(* Logix 5000 AddOnInstructionDefinition export MCFG_Yaskawa; software revision 17.00 *)

TYPE Yaskawa_EIP_Servo :   // Yaskawa SigmaLogic Axis Structure
STRUCT
   O : Yaskawa_OUT_to_Servo;
   I : Yaskawa_IN_from_Servo;
   AOI_SB : Yaskawa_AOI_Status_Bits;
END_STRUCT
END_TYPE

TYPE Yaskawa_OUT_to_Servo :   // Structure of data sent out to the Yaskawa SigmaLogic controller
STRUCT
   b00_ServoOn : BOOL;   // Servo On
   b01_Stop : BOOL;   // Stops All Current Motion in Progress
   b02_Home : BOOL;   // Start Homing Process
   b03_MoveStart1 : BOOL;   // Start Current Motion
   b06_SuperImpose : BOOL;
   b07_ServoAlarmReset : BOOL;   // Servo Alarm Reset
   b08_ControllerAlarmReset : BOOL;   // SigmaLogic Alarm Reset
   b09_MoveStart2 : BOOL;   // Start Second Motion (Blended Move)
   b10_MoveAbort : BOOL;   // Abort Current Move
   b11_MovePause : BOOL;   // Pause Current Move
   b12_SeqPause : BOOL;   // Indexing Sequence Pause
   b13_SeqResume : BOOL;   // Indexing Sequence Resume
   b14_SeqCancel : BOOL;   // Indexing Sequence Cancel
   b15_AbsEncoderReset : BOOL;   // Absolute Encoder Reset
   b16_SeqStart : BOOL;   // Start Indexing Sequence
   b17_SeqEditSpeed : BOOL;   // Enter Edit Speed
   b18_SeqEditDistance : BOOL;   // Enter Distance Edit
   b19_PLSEnable : BOOL;   // Enable PLS execution
   b20_PLSActivateOutput1 : BOOL;   // Activate PLS output1 switch logic
   b21_PLSActivateOutput2 : BOOL;   // Activate PLS output2 switch logic
   b22_PLSActivateOutput3 : BOOL;   // Activate PLS output3 switch logic
   b23_PLSActivateOutput4 : BOOL;   // Activate PLS output4 switch logic
   b24_SetClock : BOOL;   // Set the remote controller clock with data provided by the PLC
   RebootController : BOOL;
   UseExternalEncoder : BOOL;   // Use External Encoder when executing MAHSP_Yaskawa
   b32_HeatbeatAnswer : BOOL;   // Heartbeat Answer
   BrakeBypassRequest : BOOL;
   TorqueLimit : DINT;
   TorqueRamp : DINT;
   HomeMethod : INT;
   HomeSpeed : DINT;
   HomeAccDec : DINT;   // Home Move Acceleration/Deceleration Rate
   HomeBackOffDistance : DINT;
   HomeCreepSpeed : DINT;
   HomeCreepDistanceLimit : DINT;
   HomeCreepTimeLimit : DINT;
   HomeOffsetDistance : DINT;
   HomeOffsetSpeed : DINT;
   HomePostion : DINT;
   HomeTorque : DINT;
   HomeInputNo : DINT;
   HomeApproachTimeLimit : DINT;
   HomeApproachDistLimit : DINT;
   HomeDirection : INT;
   HomeSwitchMode : INT;
   MoveType : INT;
   MoveDirection : INT;
   MoveAccel1 : DINT;
   MoveAccel2 : DINT;
   MoveDecel1 : DINT;
   MoveDecel2 : DINT;
   MoveSpeed1 : DINT;
   MoveSpeed2 : DINT;
   MoveDistance1 : DINT;
   MoveDistance2 : DINT;
   MovePosition1 : DINT;
   MovePosition2 : DINT;
   RegistrationDistance : DINT;
   GearNumerator : DINT;
   GearDenominator : DINT;
   SuperImposeDistance : DINT;
   Resolution : INT;
   RegistrationDirection : INT;
   TuningLevel : INT;
   SequenceStep : INT;   // Staring Sequence Step Number
   SequenceEditStep : INT;   // Sequence Step Number to Edit
   FlagCommandBits1 : DINT;   // Flag Commands. 1..64 are General Flags, Bits 0..31 correspond to Flag 1..32
   FlagCommandBits2 : DINT;   // Flag Commands cont. 1..64 are General Flags, Bits 0..31 correspond to Flag 33..64
   DigitalOutCommandBits : DINT;   // Digital Output commands. Bits 0-7 correspond to CN13 Digital Outputs 0-7, used as Flag 73-80. Bits 8-10 correspond to CN1 Digital Outputs 0-2 used as Flag 88-90"
   SequenceEditSpeed : DINT;
   SequenceEditDistance : DINT;
   FeedRateOverride : INT;
   HSI_Enable : BOOL;
   HSI_MoveMode : BOOL;   // 0=Relative; 1=Moves per Cycle
   HSI_CalcMethod : BOOL;   // 0=Accel/Decel; 1=Time
   HSI_MoveDirection : BOOL;   // 0 = Negative; 1 = Positive
   HSI_TriggerFlag : INT;
   HSI_MovingFlag : INT;
   HSI_DwellingFlag : INT;
   HSI_DoneFlag : INT;
   HSI_MoveType : INT;   // 0=Single; 1=Repeat; 2=Repeat "x" times
   HSI_RepeatNumber : INT;
   HSI_Distance : DINT;
   HSI_Speed : DINT;
   HSI_Accel : DINT;
   HSI_MoveTime : DINT;
   HSI_DwellTime : DINT;
   PLS_OutputFlag1 : INT;
   PLS_OutputFlag2 : INT;
   PLS_OutputFlag3 : INT;
   PLS_OutputFlag4 : INT;
   PLS_OnPosition1 : DINT;
   PLS_OffPosition1 : DINT;
   PLS_OnPosition2 : DINT;
   PLS_OffPosition2 : DINT;
   PLS_OnPosition3 : DINT;
   PLS_OffPosition3 : DINT;
   PLS_OnPosition4 : DINT;
   PLS_OffPosition4 : DINT;
   PLS_OnCompensation1 : INT;
   PLS_OffCompensation1 : INT;
   PLS_OnCompensation2 : INT;
   PLS_OffCompensation2 : INT;
   PLS_OnCompensation3 : INT;
   PLS_OffCompensation3 : INT;
   PLS_OnCompensation4 : INT;
   PLS_OffCompensation4 : INT;
   RTC_Year : INT;
   RTC_Month : INT;
   RTC_Day : INT;
   RTC_Hour : INT;
   RTC_Min : INT;
   RTC_Sec : INT;
   StopDecel : DINT;
   AnalogOutput : INT;   // CN13, AO_01 [mV]
END_STRUCT
END_TYPE

TYPE Yaskawa_AOI_Status_Bits :   // Internal bits used to interlock Yaskawa AOI execution.
STRUCT
   MAM : BOOL;   // Move AOI Active
   MAJ : BOOL;   // Jog AOI Active
   MAB : BOOL;   // Blending AOI Active
   MAG : BOOL;   // Gearing AOI Active
   MAHSP : BOOL;   // Home SetPoint AOI Active
   MAH : BOOL;   // Homing AOI Active
   MSQE : BOOL;   // Sequence Edit AOI Active
   MSQR : BOOL;   // Sequence Run AOI Active
   MHSI : BOOL;   // High Speed Index AOI Active
   MSO : BOOL;   // Servo On
   MSF : BOOL;   // Servo Off
   MAFR : BOOL;   // Fault Reset
   MAS : BOOL;   // Servo Abort
   MTRQ : BOOL;   // Torque Mode Active
   MPLS : BOOL;   // PLS Active
   MCLK : BOOL;   // SetClock Active
   AOI_Permissive : BOOL;   // Permissive to Execute an AOI
END_STRUCT
END_TYPE

TYPE Yaskawa_IN_from_Servo :   // Structure of data coming from the Yaskawa SigmaLogic controller.
STRUCT
   AlarmText : STRING;   // ServoPack Alarm Code plus Text Description
   b00_Heartbeat : BOOL;
   b01_Alarm : BOOL;   // ServoPack Alarm
   b02_Warning : BOOL;   // ServoPack Warning
   b03_Ready : BOOL;   // ServoPack Ready
   b04_Enabled : BOOL;   // ServoPack Enabled ("Servo On")
   b05_StopComplete : BOOL;
   b06_HomeComplete : BOOL;
   b07_HomeBusy : BOOL;
   b08_HomeActive : BOOL;
   b09_HomeAborted : BOOL;
   b10_HomeError : BOOL;
   b11_MoveAbsComplete : BOOL;
   b12_MoveAbsBusy : BOOL;
   b13_MoveAbsActive : BOOL;
   b14_MoveAbsAborted : BOOL;
   b15_MoveAbsError : BOOL;
   b16_MoveRelComplete : BOOL;
   b17_MoveRelBusy : BOOL;
   b18_MoveRelActive : BOOL;
   b19_MoveRelAborted : BOOL;
   b20_MoveRelError : BOOL;
   b21_JogAtSpeed : BOOL;
   b22_JogBusy : BOOL;
   b23_JogActive : BOOL;
   b24_JogAborted : BOOL;
   b25_JogError : BOOL;
   b26_GearInSync : BOOL;
   b27_GearBusy : BOOL;
   b28_GearActive : BOOL;
   b29_GearAborted : BOOL;
   b30_GearError : BOOL;
   b32_MoveSuperComplete : BOOL;
   b33_MoveSuperBusy : BOOL;
   b34_MoveSuperActive : BOOL;
   b35_MoveSuperAborted : BOOL;
   b36_MoveSuperError : BOOL;
   b37_PowerCycleRequired : BOOL;
   b38_MoveBlend1Complete : BOOL;
   b39_MoveBlend1Busy : BOOL;
   b40_MoveBlend1Active : BOOL;
   b41_MoveBlend1Abort : BOOL;
   b42_MoveBlend1Error : BOOL;
   b43_MoveBlend2Complete : BOOL;
   b44_MoveBlend2Busy : BOOL;
   b45_MoveBlend2Active : BOOL;
   b46_MoveBlend2Abort : BOOL;
   b47_MoveBlend2Error : BOOL;
   b48_RegComplete : BOOL;
   b49_RegBusy : BOOL;
   b50_RegActive : BOOL;
   b51_RegAborted : BOOL;
   b52_RegError : BOOL;
   b53_ResetAbsEncoderActive : BOOL;
   b54_ResetAbsEncoderBusy : BOOL;
   b55_ResetAbsEncoderDone : BOOL;
   b56_ResetAbsEncoderError : BOOL;
   b57_SeqRunning : BOOL;
   b58_RegSensorNotReached : BOOL;
   b59_SeqEditError : BOOL;
   b60_SeqEditDone : BOOL;
   b61_TorqueAtTorque : BOOL;
   b62_TorqueBusy : BOOL;
   b63_TorqueActive : BOOL;
   b64_TorqueAborted : BOOL;
   b65_TorqueError : BOOL;
   b66_ControllerAlarm : BOOL;
   b67_ApplicationError : BOOL;
   b68_AxisAtStandStill : BOOL;
   b69_TestModeActive : BOOL;
   b70_ServoParamsOK : BOOL;
   Position : DINT;
   Speed : DINT;
   Torque : DINT;
   HomeErrorID : INT;
   MoveAbsErrorID : INT;
   MoveRelErrorID : INT;
   JogErrorID : INT;
   GearErrorID : INT;
   MoveSuperErrorID : INT;
   ServoAlarmID : INT;
   ServoWarningID : INT;
   ControllerAlarmID : DINT;
   AxisGenAlarmID : DINT;
   MoveBlend1ErrorID : INT;
   MoveBlend2ErrorID : INT;
   ResetAbsEncoderErrorID : INT;
   FunctionBlockErrorID : INT;
   TorqueErrorID : INT;
   RegErrorID : INT;
   SeqCurrentStep : INT;
   FlagStatusBit1 : DINT;   // Flag Status. 1..64 are General Flags, Bits 0..31 correspond to Flag 1..32
   FlagStatusBit2 : DINT;   // Flag Status cont. 1..64 are General Flags, Bits 0..31 correspond to Flag 33..64
   IOStatusBits : DINT;   // Digital IO Status. Bits 0-7, CN13 Inputs 0-7, Used as Flag 65-72. Bits 8-15, CN13 Outputs 0-7, Used as Flag 73-80. Bits 16-22, CN1 Inputs 0-6, Used as Flag 81-87. Bits 23-25, CN1 Outputs 0-2, Used as Flag 88-90.
   HSI_Moving : BOOL;
   HSI_Dwelling : BOOL;
   HSI_Done : BOOL;
   HSI_Busy : BOOL;
   HSI_Error : BOOL;
   HSI_ErrorCode : INT;
   PLS_Running : BOOL;
   PLS_SwitchStatus1 : BOOL;
   PLS_SwitchStatus2 : BOOL;
   PLS_SwitchStatus3 : BOOL;
   PLS_SwitchStatus4 : BOOL;
   PLS_Busy : BOOL;
   PLS_Error : BOOL;
   PLS_ErrorCode : INT;
   SetClock_Done : BOOL;
   SetClock_Busy : BOOL;
   SetClock_Error : BOOL;
   SetClock_ErrorID : INT;
   SoftwareVersion : DINT;
   FirmwareVersion : DINT;
   CommandedPos : DINT;
   CommandedPosNonCyc : DINT;
   CommandedSpeed : DINT;
   Clock_Year : INT;
   Clock_Month : INT;
   Clock_Day : INT;
   Clock_Hour : INT;
   Clock_Minute : INT;
   Clock_Second : INT;
   AnalogInput : REAL;   // CN13, AI_01 [v]
   BrakeBypassActive : BOOL;
END_STRUCT
END_TYPE

ADD_ON_INSTRUCTION MCFG_Yaskawa   (* revision 2.0 0, vendor Yaskawa America, Inc., ExecutePrescan *)
// Motion Axis Configuration & Status
// Revision note:
// 2.0.0: Adds mapping for brake override and rebooting controller. Adds MotionIdle and HomingIdle outputs. Moves Alarm text parsing from MCFG to new MRSE instruction. Adds RegErrorID to inputs. Adds outputs for ExternalEncoder position and speed.
// 1.2.0: Adds mapping for Analog Output and analog Output.
// Detectsl mismatches between AOI version and SigmaLogic software version.
// Requires updated DataTypes for Yaskawa_IN_from_Servo and Yaskawa_EIP_Servo.
// 1.1.0: Initial Release 9/10/2014
// Help:
// This AOI handles all the 'packing' and 'unpacking' of motion command tag data into the Ethernet instances for communication between the PLC and SigmaLogic axis. It is the only REQUIRED AOI to ensure functionality.
// All essential axis information can be found at this AOI including axis Position, Speed, Torque, Error Codes and Software/Firmware versions.
// Internally, this AOI monitors a 'Heatbeat' input data point from the attached SigmaLogic axis. This heartbeat signal is internally reflected by the MCFG_Yaskawa AOI to the output instance and can be monitored by the application code. The SigmaLogic monitors the reflected signal from the PLC and the servo will be held in a disabled state if it is not present. The duty cycle of the heartbeat signal is approx. 0.5 sec ON and 0.5 sec OFF.
// Feedrate override can be adjusted between 1-200% of the programmed speed for the selected move. If left at default of 0 and never changed, the actual feedrate will be set at 100%. Once the override is set between 1 and 200, the setting will always be active. For MAJ_Yaskawa command (Motion Axis Jog),  changes to feedrate override will take effect immediately. For all other commanded moves, changes will take effect at the beginning of the next move.
// Starting in v2.0.x new outputs were added for MotionIdle and HomingIdle. These outputs are available for interlocking purposes and indicate when the SigmaLogic axis is ready to start new motion (execute the next Motion or Homing AOI).
// Feedrate override can be adjusted between 1-200% of the programmed speed for the selected move. If left at default of 0 and never changed, the actual feedrate will be set at 100%. Once the override is set between 1 and 200, the setting will always be active. For MAJ_Yaskawa command (Motion Axis Jog),  changes to feedrate override will take effect immediately. For all other commanded moves, changes will take effect at the beginning of the next move.
VAR_IN_OUT
   Axis_IN : AB:ETHERNET_MODULE_DINT_256Bytes:I:0; {required}
   Axis_OUT : AB:ETHERNET_MODULE_DINT_256Bytes:O:0; {required}
   Axis : Yaskawa_EIP_Servo; {required}
END_VAR
VAR_INPUT
   ParameterResolution : INT; {required}   // Desired decimal places for Real Numbers
   FeedRateOverride : INT := 100; {required}   // Speed Override: 1% - 200% (100% = programmed speed)
END_VAR
VAR_OUTPUT
   PositionFB : REAL; {visible}   // Actual Position Feedback
   SpeedFB : REAL; {visible}   // Actual Speed Feedback
   TorqueFB : REAL; {visible}   // Actual Torque Feedback
   ExtPositionFB : REAL; {visible}   // Actual Position Feedback of the External Encoder
   ExtSpeedFB : REAL; {visible}   // Actual Speed Feedback of the External Encoder
   ServoAlarmCode : INT; {visible}   // Servo Alarm Code
   ServoWarningCode : INT; {visible}   // Servo Warning Code
   ControllerAlarmCode : DINT; {visible}   // Controller Alarm Code
   ApplicationErrorCode : INT; {visible}   // Application Function Block Error Code
   EN : BOOL; {visible}
   HB : BOOL; {visible}   // Heartbeaat pulse from SigmaLogic axis.
   CommFLT : BOOL; {visible}   // Communication Fault. Heartbeat was lost.
   MotionIdle : BOOL; {visible}   // Indicates that the Axis is ready to accept a new motion command
   HomingIdle : BOOL; {visible}   // Indicates that the Axis is ready to accept a new homing command
   SvPrmOK : BOOL; {visible}   // Servo parameters have been successfully downloaded and confirmed
   SvRDY : BOOL; {visible}   // Servo Ready
   SvON : BOOL; {visible}   // Servo On
   SvSTL : BOOL; {visible}   // Servo is at StandStill according to the PLCopen Motion State Model and has finished executing any motion commands. Use this output in combination with MotionIdle and/or HomingIdle to interlock when a new motion command can be started.
   SvALM : BOOL; {visible}   // Servo Alarm
   SvWRN : BOOL; {visible}   // Servo Warning
   SvABT : BOOL; {visible}   // Servo Move Aborted
   CntrALM : BOOL; {visible}   // Controller Alarm is present
   AppER : BOOL; {visible}   // An Application error is present
   AOI_Active : BOOL; {visible}   // An Axis AOI is Active
   SigmaLogicSoftware : DINT; {visible}   // Software version of embedded code installed in the SigmaLogic controller.
   SigmaLogicFirmware : DINT; {visible}   // Firmware version installed in the SigmaLogic Controller
   TestMode : BOOL; {visible}   // Test Mode set by Configuration Utility is Active. PLC control is blocked
   SftwreMismatch : BOOL; {visible}   // A mismatch between the AOI version and the SigmaLogic Software version has been detected. Check the compatability table at www.yaskawa.com/sigmalogic.
END_VAR
VAR
   PermissiveAssist1 : BOOL;
   PermissiveAssist2 : BOOL;
   PermissiveAssist3 : BOOL;
   ScaleFactor : DINT;
   Enabled_OSF : BOOL;   // One-Shot that detects the falling Edge of the Enabled Status.
   AlwaysOFF : BOOL;
   OneShot0 : BOOL;
   HB_T1 : TIMER := (PRE := 750);
   HB_T2 : TIMER := (PRE := 750);
   OneShot1 : BOOL;
   tempAO : INT;
   AOIversion : INT;   // Version number of the main AOI Release, mainly tracked in the version of MCFG_Yaskawa.
END_VAR

ROUTINE Logic   (* ladder *)
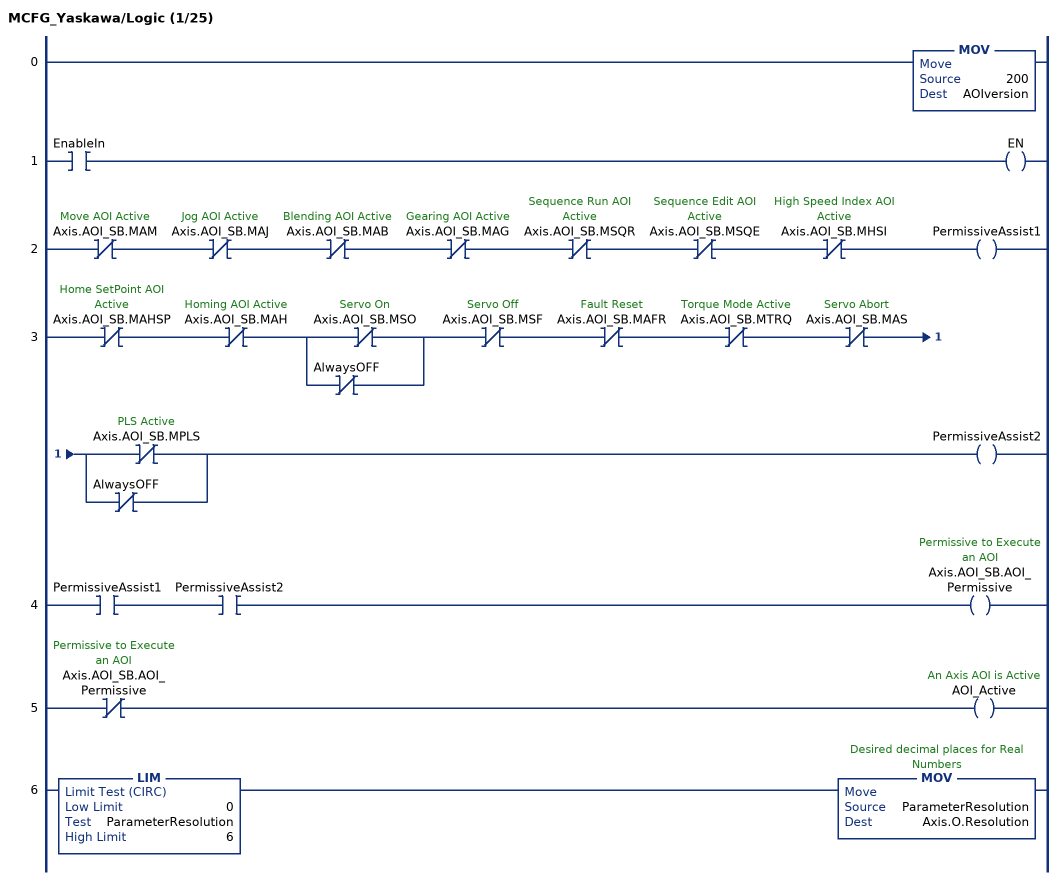
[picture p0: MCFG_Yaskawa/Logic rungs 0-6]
   0: MOV(200,AOIversion);
   1: XIC(EnableIn)OTE(EN);
   2: XIO(Axis.AOI_SB.MAM)XIO(Axis.AOI_SB.MAJ)XIO(Axis.AOI_SB.MAB)XIO(Axis.AOI_SB.MAG)XIO(Axis.AOI_SB.MSQR)XIO(Axis.AOI_SB.MSQE)XIO(Axis.AOI_SB.MHSI)OTE(PermissiveAssist1);
   3: XIO(Axis.AOI_SB.MAHSP)XIO(Axis.AOI_SB.MAH)[XIO(Axis.AOI_SB.MSO) ,XIO(AlwaysOFF) ]XIO(Axis.AOI_SB.MSF)XIO(Axis.AOI_SB.MAFR)XIO(Axis.AOI_SB.MTRQ)XIO(Axis.AOI_SB.MAS)[XIO(Axis.AOI_SB.MPLS) ,XIO(AlwaysOFF) ]OTE(PermissiveAssist2);
   4: XIC(PermissiveAssist1)XIC(PermissiveAssist2)OTE(Axis.AOI_SB.AOI_Permissive);
   5: XIO(Axis.AOI_SB.AOI_Permissive)OTE(AOI_Active);
   6: LIM(0,ParameterResolution,6)MOV(ParameterResolution,Axis.O.Resolution);
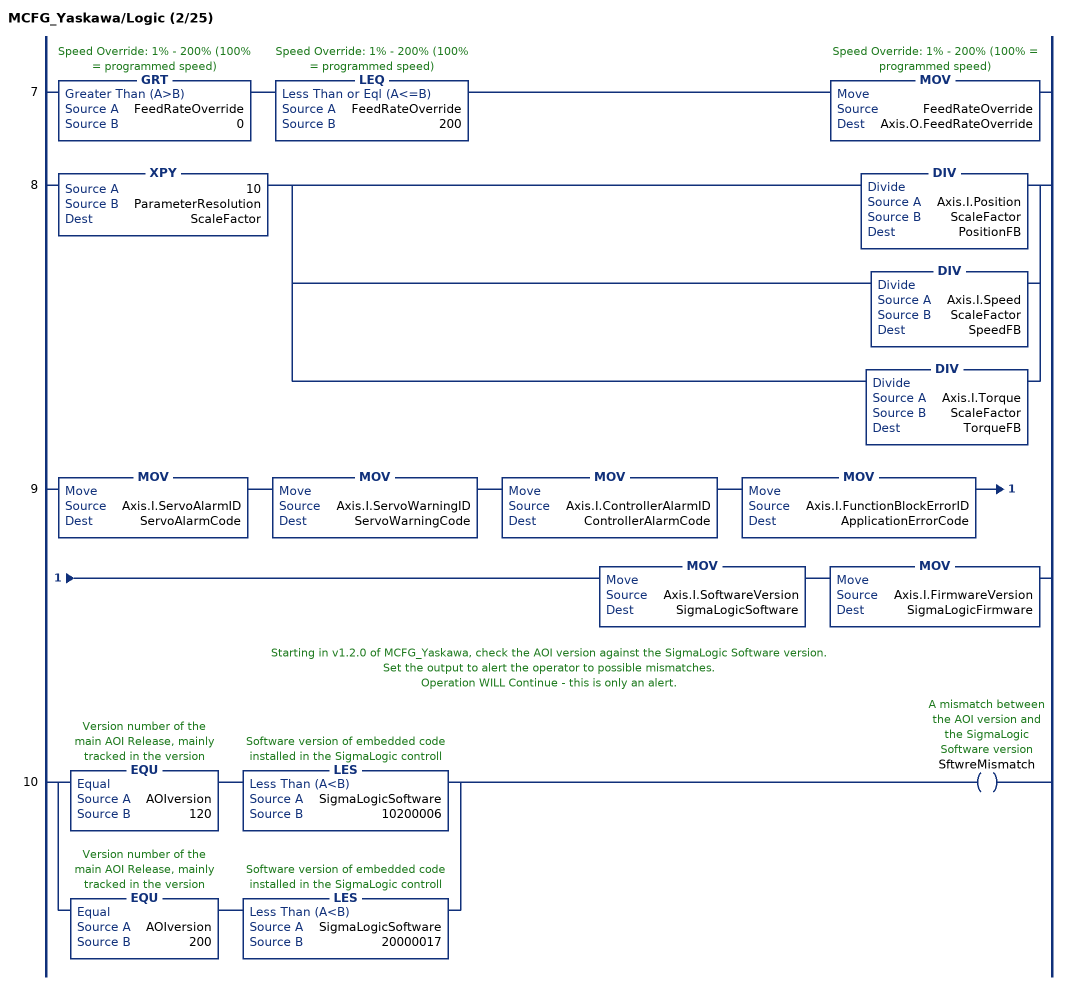
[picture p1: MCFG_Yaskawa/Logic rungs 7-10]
   7: GRT(FeedRateOverride,0)LEQ(FeedRateOverride,200)MOV(FeedRateOverride,Axis.O.FeedRateOverride);
   8: XPY(10,ParameterResolution,ScaleFactor)[DIV(Axis.I.Position,ScaleFactor,PositionFB) ,DIV(Axis.I.Speed,ScaleFactor,SpeedFB) ,DIV(Axis.I.Torque,ScaleFactor,TorqueFB) ];
   9: MOV(Axis.I.ServoAlarmID,ServoAlarmCode)MOV(Axis.I.ServoWarningID,ServoWarningCode)MOV(Axis.I.ControllerAlarmID,ControllerAlarmCode)MOV(Axis.I.FunctionBlockErrorID,ApplicationErrorCode)MOV(Axis.I.SoftwareVersion,SigmaLogicSoftware)MOV(Axis.I.FirmwareVersion,SigmaLogicFirmware);
   // Starting in v1.2.0 of MCFG_Yaskawa, check the AOI version against the SigmaLogic Software version.
   // Set the output to alert the operator to possible mismatches.
   // Operation WILL Continue - this is only an alert.
   10: [EQU(AOIversion,120) LES(SigmaLogicSoftware,10200006) ,EQU(AOIversion,200) LES(SigmaLogicSoftware,20000017) ]OTE(SftwreMismatch);
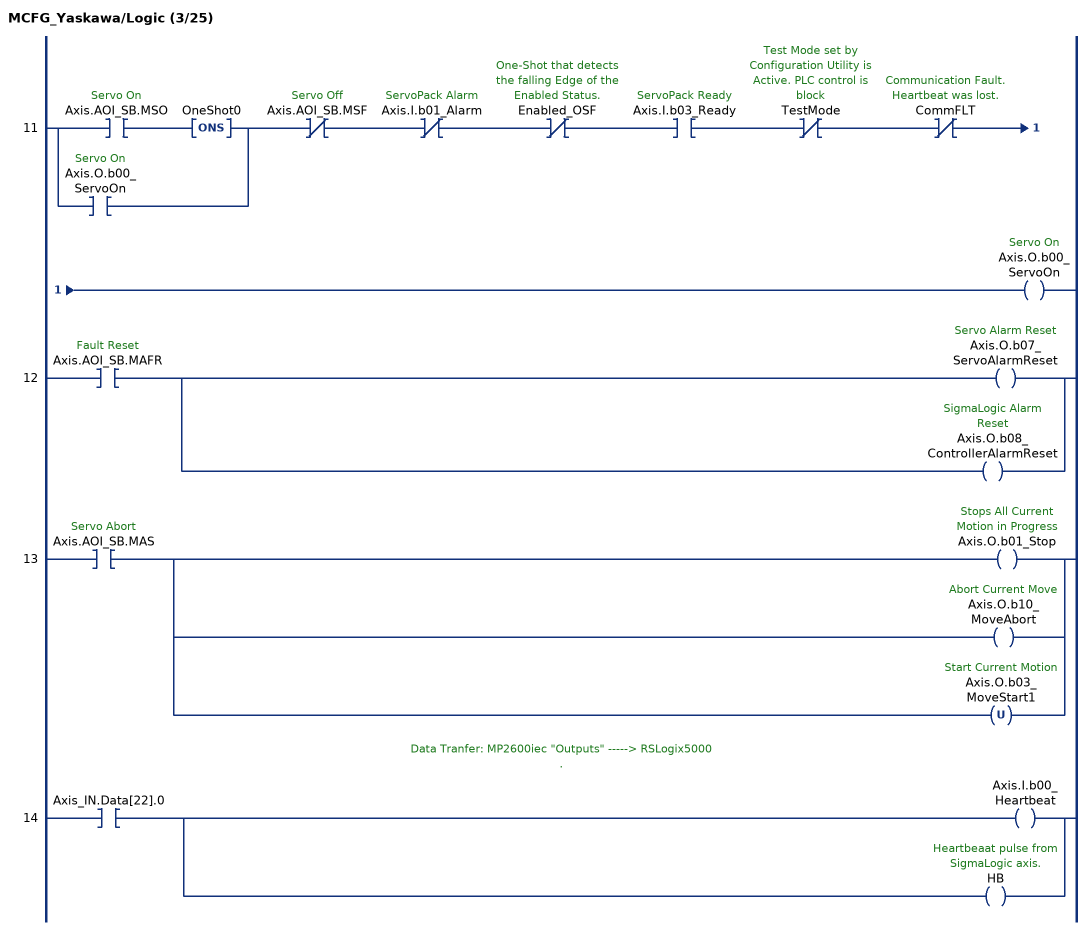
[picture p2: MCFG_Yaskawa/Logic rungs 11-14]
   11: [XIC(Axis.AOI_SB.MSO) ONS(OneShot0) ,XIC(Axis.O.b00_ServoOn) ]XIO(Axis.AOI_SB.MSF)XIO(Axis.I.b01_Alarm)XIO(Enabled_OSF)XIC(Axis.I.b03_Ready)XIO(TestMode)XIO(CommFLT)OTE(Axis.O.b00_ServoOn);
   12: XIC(Axis.AOI_SB.MAFR)[OTE(Axis.O.b07_ServoAlarmReset) ,OTE(Axis.O.b08_ControllerAlarmReset) ];
   13: XIC(Axis.AOI_SB.MAS)[OTE(Axis.O.b01_Stop) ,OTE(Axis.O.b10_MoveAbort) ,OTU(Axis.O.b03_MoveStart1) ];
   // Data Tranfer: MP2600iec "Outputs" -----> RSLogix5000
   // .
   14: XIC(Axis_IN.Data[22].0)[OTE(Axis.I.b00_Heartbeat) ,OTE(HB) ];
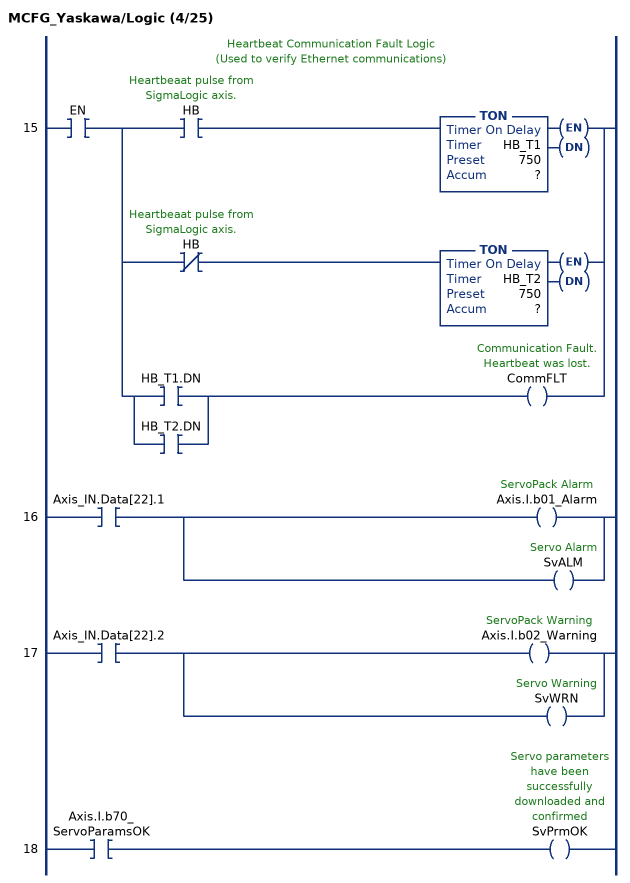
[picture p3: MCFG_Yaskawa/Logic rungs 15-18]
   // Heartbeat Communication Fault Logic
   // (Used to verify Ethernet communications)
   15: XIC(EN)[XIC(HB) TON(HB_T1,?,?) ,XIO(HB) TON(HB_T2,?,?) ,[XIC(HB_T1.DN) ,XIC(HB_T2.DN) ] OTE(CommFLT) ];
   16: XIC(Axis_IN.Data[22].1)[OTE(Axis.I.b01_Alarm) ,OTE(SvALM) ];
   17: XIC(Axis_IN.Data[22].2)[OTE(Axis.I.b02_Warning) ,OTE(SvWRN) ];
   18: XIC(Axis.I.b70_ServoParamsOK)OTE(SvPrmOK);
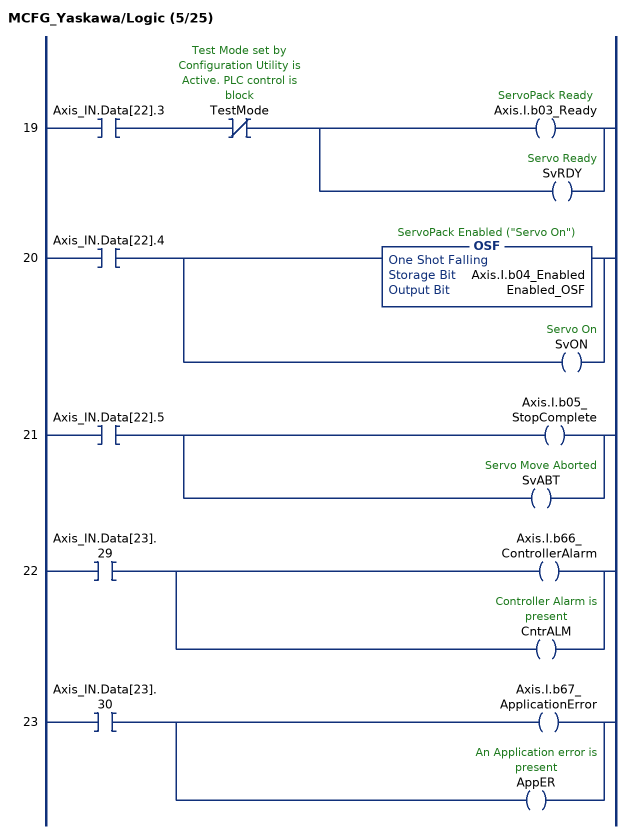
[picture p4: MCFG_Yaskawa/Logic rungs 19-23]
   19: XIC(Axis_IN.Data[22].3)XIO(TestMode)[OTE(Axis.I.b03_Ready) ,OTE(SvRDY) ];
   20: XIC(Axis_IN.Data[22].4)[OSF(Axis.I.b04_Enabled,Enabled_OSF) ,OTE(SvON) ];
   21: XIC(Axis_IN.Data[22].5)[OTE(Axis.I.b05_StopComplete) ,OTE(SvABT) ];
   22: XIC(Axis_IN.Data[23].29)[OTE(Axis.I.b66_ControllerAlarm) ,OTE(CntrALM) ];
   23: XIC(Axis_IN.Data[23].30)[OTE(Axis.I.b67_ApplicationError) ,OTE(AppER) ];
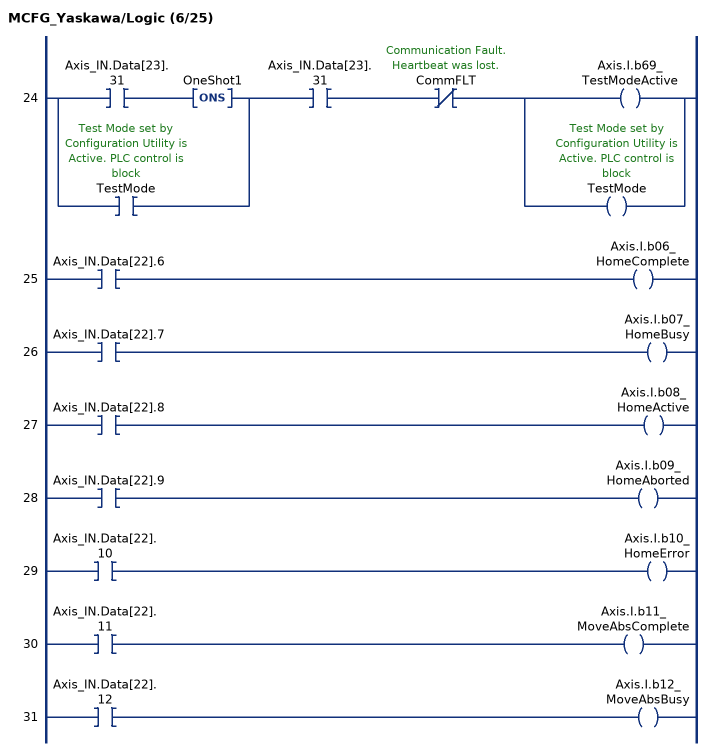
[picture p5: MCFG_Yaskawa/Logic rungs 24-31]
   24: [XIC(Axis_IN.Data[23].31) ONS(OneShot1) ,XIC(TestMode) ]XIC(Axis_IN.Data[23].31)XIO(CommFLT)[OTE(Axis.I.b69_TestModeActive) ,OTE(TestMode) ];
   25: XIC(Axis_IN.Data[22].6)OTE(Axis.I.b06_HomeComplete);
   26: XIC(Axis_IN.Data[22].7)OTE(Axis.I.b07_HomeBusy);
   27: XIC(Axis_IN.Data[22].8)OTE(Axis.I.b08_HomeActive);
   28: XIC(Axis_IN.Data[22].9)OTE(Axis.I.b09_HomeAborted);
   29: XIC(Axis_IN.Data[22].10)OTE(Axis.I.b10_HomeError);
   30: XIC(Axis_IN.Data[22].11)OTE(Axis.I.b11_MoveAbsComplete);
   31: XIC(Axis_IN.Data[22].12)OTE(Axis.I.b12_MoveAbsBusy);
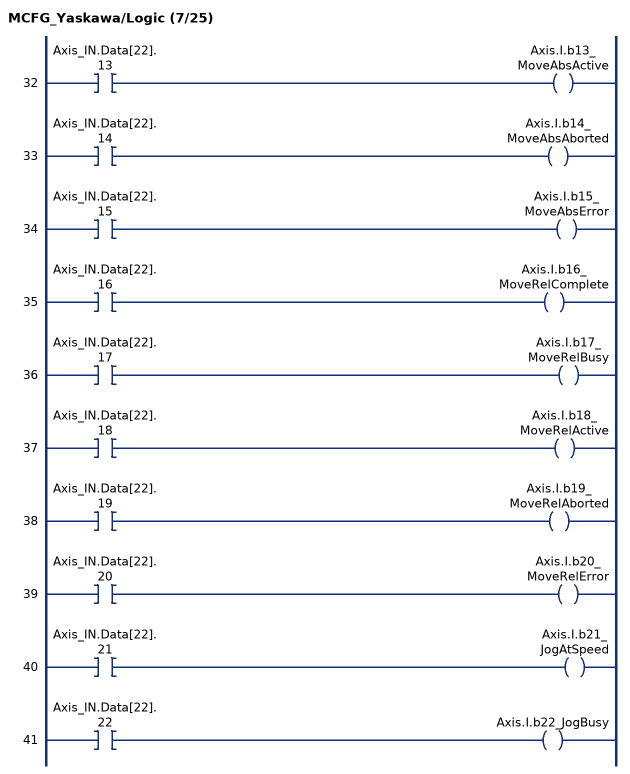
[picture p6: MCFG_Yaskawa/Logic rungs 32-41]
   32: XIC(Axis_IN.Data[22].13)OTE(Axis.I.b13_MoveAbsActive);
   33: XIC(Axis_IN.Data[22].14)OTE(Axis.I.b14_MoveAbsAborted);
   34: XIC(Axis_IN.Data[22].15)OTE(Axis.I.b15_MoveAbsError);
   35: XIC(Axis_IN.Data[22].16)OTE(Axis.I.b16_MoveRelComplete);
   36: XIC(Axis_IN.Data[22].17)OTE(Axis.I.b17_MoveRelBusy);
   37: XIC(Axis_IN.Data[22].18)OTE(Axis.I.b18_MoveRelActive);
   38: XIC(Axis_IN.Data[22].19)OTE(Axis.I.b19_MoveRelAborted);
   39: XIC(Axis_IN.Data[22].20)OTE(Axis.I.b20_MoveRelError);
   40: XIC(Axis_IN.Data[22].21)OTE(Axis.I.b21_JogAtSpeed);
   41: XIC(Axis_IN.Data[22].22)OTE(Axis.I.b22_JogBusy);
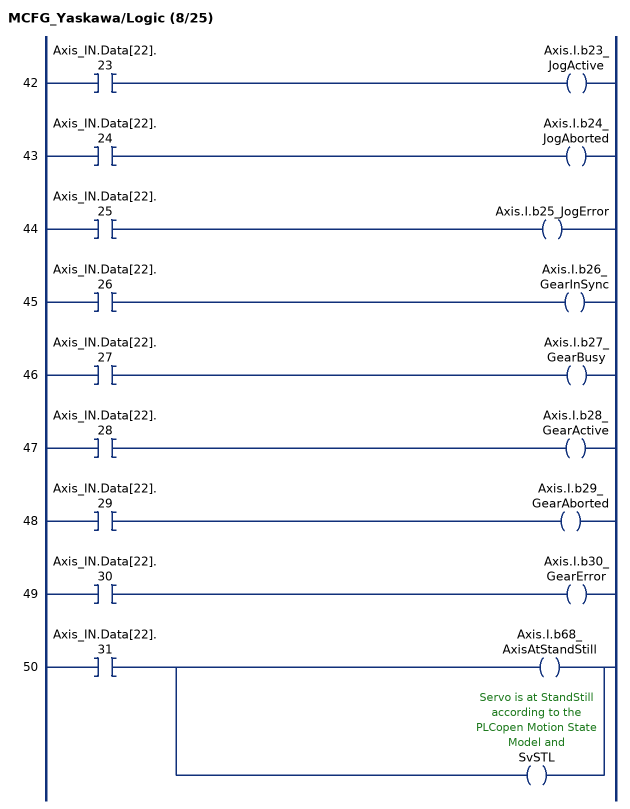
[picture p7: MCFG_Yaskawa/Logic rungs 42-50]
   42: XIC(Axis_IN.Data[22].23)OTE(Axis.I.b23_JogActive);
   43: XIC(Axis_IN.Data[22].24)OTE(Axis.I.b24_JogAborted);
   44: XIC(Axis_IN.Data[22].25)OTE(Axis.I.b25_JogError);
   45: XIC(Axis_IN.Data[22].26)OTE(Axis.I.b26_GearInSync);
   46: XIC(Axis_IN.Data[22].27)OTE(Axis.I.b27_GearBusy);
   47: XIC(Axis_IN.Data[22].28)OTE(Axis.I.b28_GearActive);
   48: XIC(Axis_IN.Data[22].29)OTE(Axis.I.b29_GearAborted);
   49: XIC(Axis_IN.Data[22].30)OTE(Axis.I.b30_GearError);
   50: XIC(Axis_IN.Data[22].31)[OTE(Axis.I.b68_AxisAtStandStill) ,OTE(SvSTL) ];
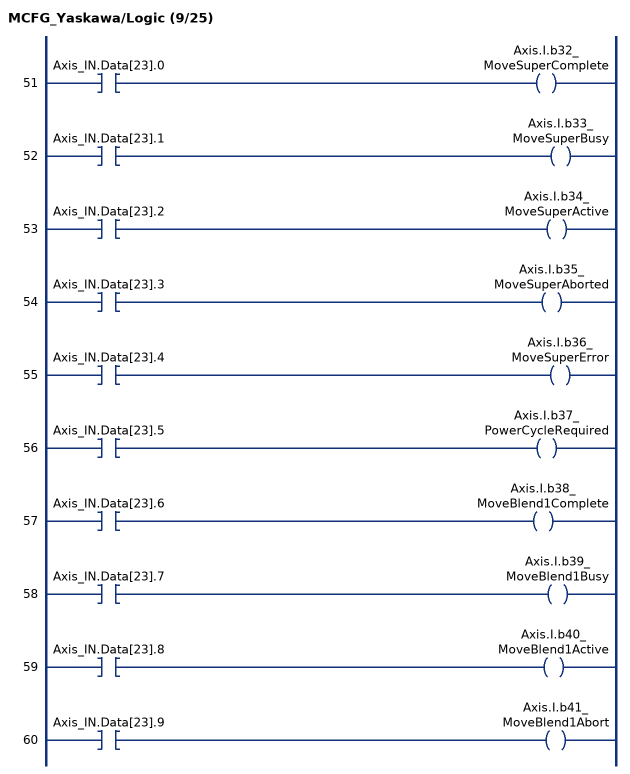
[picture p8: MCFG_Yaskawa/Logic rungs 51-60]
   51: XIC(Axis_IN.Data[23].0)OTE(Axis.I.b32_MoveSuperComplete);
   52: XIC(Axis_IN.Data[23].1)OTE(Axis.I.b33_MoveSuperBusy);
   53: XIC(Axis_IN.Data[23].2)OTE(Axis.I.b34_MoveSuperActive);
   54: XIC(Axis_IN.Data[23].3)OTE(Axis.I.b35_MoveSuperAborted);
   55: XIC(Axis_IN.Data[23].4)OTE(Axis.I.b36_MoveSuperError);
   56: XIC(Axis_IN.Data[23].5)OTE(Axis.I.b37_PowerCycleRequired);
   57: XIC(Axis_IN.Data[23].6)OTE(Axis.I.b38_MoveBlend1Complete);
   58: XIC(Axis_IN.Data[23].7)OTE(Axis.I.b39_MoveBlend1Busy);
   59: XIC(Axis_IN.Data[23].8)OTE(Axis.I.b40_MoveBlend1Active);
   60: XIC(Axis_IN.Data[23].9)OTE(Axis.I.b41_MoveBlend1Abort);
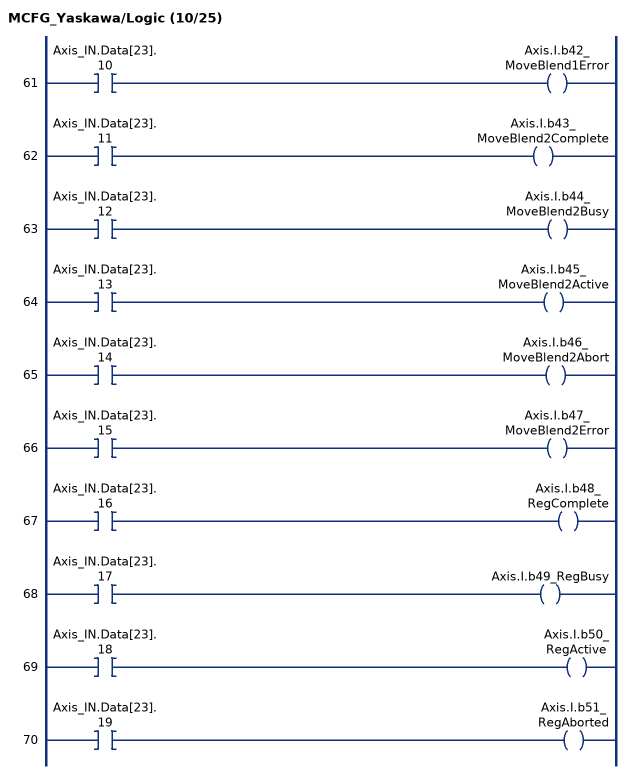
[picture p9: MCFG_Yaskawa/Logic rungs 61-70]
   61: XIC(Axis_IN.Data[23].10)OTE(Axis.I.b42_MoveBlend1Error);
   62: XIC(Axis_IN.Data[23].11)OTE(Axis.I.b43_MoveBlend2Complete);
   63: XIC(Axis_IN.Data[23].12)OTE(Axis.I.b44_MoveBlend2Busy);
   64: XIC(Axis_IN.Data[23].13)OTE(Axis.I.b45_MoveBlend2Active);
   65: XIC(Axis_IN.Data[23].14)OTE(Axis.I.b46_MoveBlend2Abort);
   66: XIC(Axis_IN.Data[23].15)OTE(Axis.I.b47_MoveBlend2Error);
   67: XIC(Axis_IN.Data[23].16)OTE(Axis.I.b48_RegComplete);
   68: XIC(Axis_IN.Data[23].17)OTE(Axis.I.b49_RegBusy);
   69: XIC(Axis_IN.Data[23].18)OTE(Axis.I.b50_RegActive);
   70: XIC(Axis_IN.Data[23].19)OTE(Axis.I.b51_RegAborted);
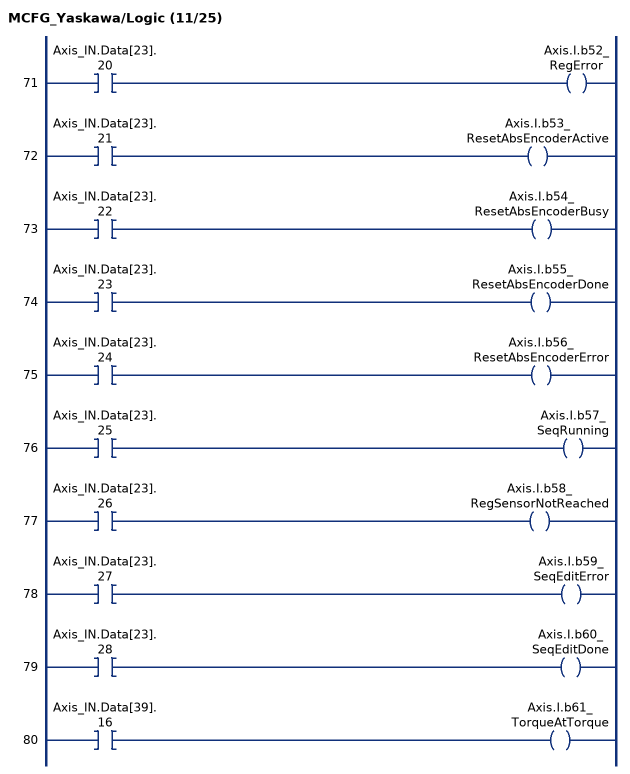
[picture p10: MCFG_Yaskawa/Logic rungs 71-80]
   71: XIC(Axis_IN.Data[23].20)OTE(Axis.I.b52_RegError);
   72: XIC(Axis_IN.Data[23].21)OTE(Axis.I.b53_ResetAbsEncoderActive);
   73: XIC(Axis_IN.Data[23].22)OTE(Axis.I.b54_ResetAbsEncoderBusy);
   74: XIC(Axis_IN.Data[23].23)OTE(Axis.I.b55_ResetAbsEncoderDone);
   75: XIC(Axis_IN.Data[23].24)OTE(Axis.I.b56_ResetAbsEncoderError);
   76: XIC(Axis_IN.Data[23].25)OTE(Axis.I.b57_SeqRunning);
   77: XIC(Axis_IN.Data[23].26)OTE(Axis.I.b58_RegSensorNotReached);
   78: XIC(Axis_IN.Data[23].27)OTE(Axis.I.b59_SeqEditError);
   79: XIC(Axis_IN.Data[23].28)OTE(Axis.I.b60_SeqEditDone);
   80: XIC(Axis_IN.Data[39].16)OTE(Axis.I.b61_TorqueAtTorque);
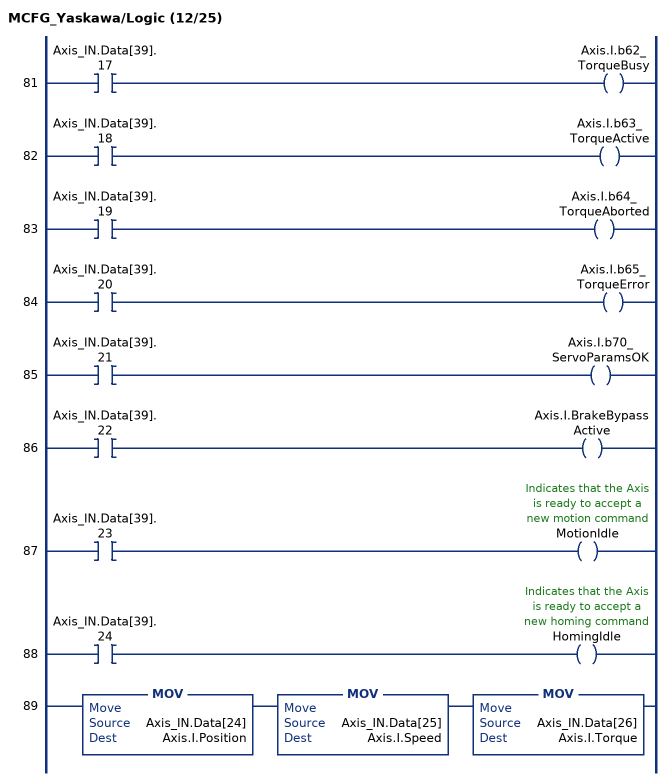
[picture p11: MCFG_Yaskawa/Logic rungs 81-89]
   81: XIC(Axis_IN.Data[39].17)OTE(Axis.I.b62_TorqueBusy);
   82: XIC(Axis_IN.Data[39].18)OTE(Axis.I.b63_TorqueActive);
   83: XIC(Axis_IN.Data[39].19)OTE(Axis.I.b64_TorqueAborted);
   84: XIC(Axis_IN.Data[39].20)OTE(Axis.I.b65_TorqueError);
   85: XIC(Axis_IN.Data[39].21)OTE(Axis.I.b70_ServoParamsOK);
   86: XIC(Axis_IN.Data[39].22)OTE(Axis.I.BrakeBypassActive);
   87: XIC(Axis_IN.Data[39].23)OTE(MotionIdle);
   88: XIC(Axis_IN.Data[39].24)OTE(HomingIdle);
   89: MOV(Axis_IN.Data[24],Axis.I.Position)MOV(Axis_IN.Data[25],Axis.I.Speed)MOV(Axis_IN.Data[26],Axis.I.Torque);
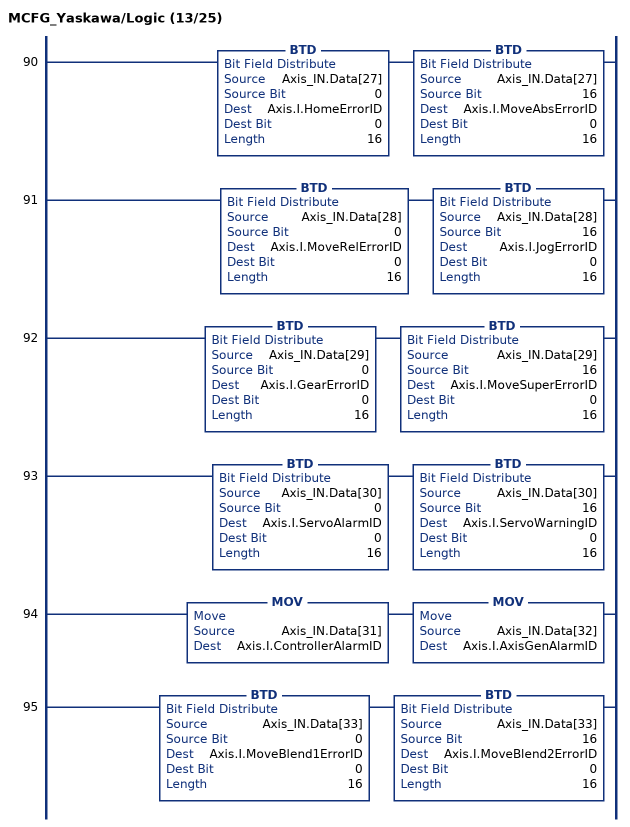
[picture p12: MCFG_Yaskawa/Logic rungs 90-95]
   90: BTD(Axis_IN.Data[27],0,Axis.I.HomeErrorID,0,16)BTD(Axis_IN.Data[27],16,Axis.I.MoveAbsErrorID,0,16);
   91: BTD(Axis_IN.Data[28],0,Axis.I.MoveRelErrorID,0,16)BTD(Axis_IN.Data[28],16,Axis.I.JogErrorID,0,16);
   92: BTD(Axis_IN.Data[29],0,Axis.I.GearErrorID,0,16)BTD(Axis_IN.Data[29],16,Axis.I.MoveSuperErrorID,0,16);
   93: BTD(Axis_IN.Data[30],0,Axis.I.ServoAlarmID,0,16)BTD(Axis_IN.Data[30],16,Axis.I.ServoWarningID,0,16);
   94: MOV(Axis_IN.Data[31],Axis.I.ControllerAlarmID)MOV(Axis_IN.Data[32],Axis.I.AxisGenAlarmID);
   95: BTD(Axis_IN.Data[33],0,Axis.I.MoveBlend1ErrorID,0,16)BTD(Axis_IN.Data[33],16,Axis.I.MoveBlend2ErrorID,0,16);
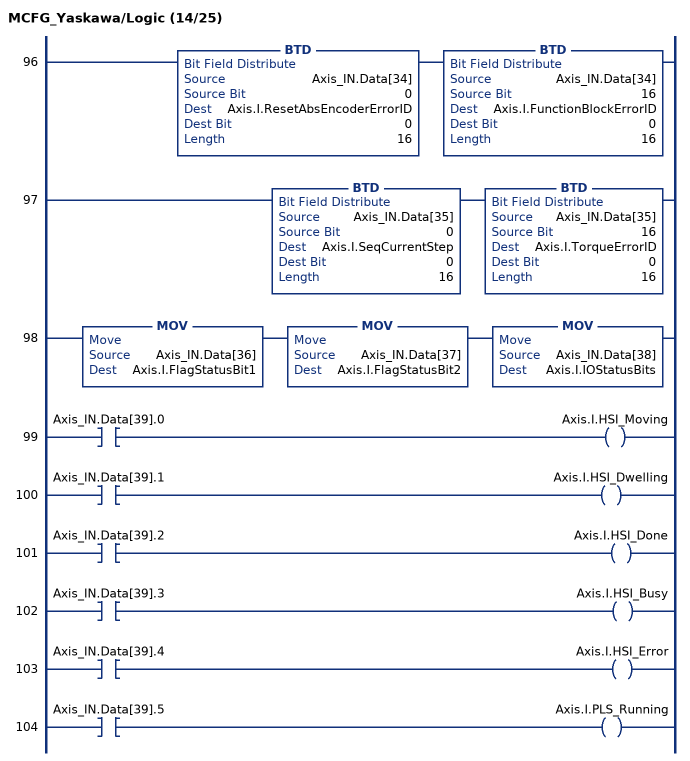
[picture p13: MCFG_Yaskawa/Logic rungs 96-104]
   96: BTD(Axis_IN.Data[34],0,Axis.I.ResetAbsEncoderErrorID,0,16)BTD(Axis_IN.Data[34],16,Axis.I.FunctionBlockErrorID,0,16);
   97: BTD(Axis_IN.Data[35],0,Axis.I.SeqCurrentStep,0,16)BTD(Axis_IN.Data[35],16,Axis.I.TorqueErrorID,0,16);
   98: MOV(Axis_IN.Data[36],Axis.I.FlagStatusBit1)MOV(Axis_IN.Data[37],Axis.I.FlagStatusBit2)MOV(Axis_IN.Data[38],Axis.I.IOStatusBits);
   99: XIC(Axis_IN.Data[39].0)OTE(Axis.I.HSI_Moving);
   100: XIC(Axis_IN.Data[39].1)OTE(Axis.I.HSI_Dwelling);
   101: XIC(Axis_IN.Data[39].2)OTE(Axis.I.HSI_Done);
   102: XIC(Axis_IN.Data[39].3)OTE(Axis.I.HSI_Busy);
   103: XIC(Axis_IN.Data[39].4)OTE(Axis.I.HSI_Error);
   104: XIC(Axis_IN.Data[39].5)OTE(Axis.I.PLS_Running);
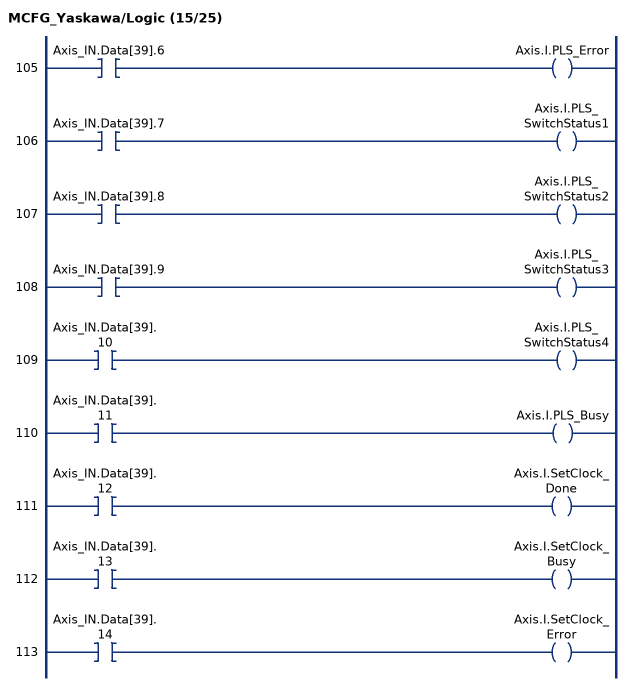
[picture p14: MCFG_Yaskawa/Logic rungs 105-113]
   105: XIC(Axis_IN.Data[39].6)OTE(Axis.I.PLS_Error);
   106: XIC(Axis_IN.Data[39].7)OTE(Axis.I.PLS_SwitchStatus1);
   107: XIC(Axis_IN.Data[39].8)OTE(Axis.I.PLS_SwitchStatus2);
   108: XIC(Axis_IN.Data[39].9)OTE(Axis.I.PLS_SwitchStatus3);
   109: XIC(Axis_IN.Data[39].10)OTE(Axis.I.PLS_SwitchStatus4);
   110: XIC(Axis_IN.Data[39].11)OTE(Axis.I.PLS_Busy);
   111: XIC(Axis_IN.Data[39].12)OTE(Axis.I.SetClock_Done);
   112: XIC(Axis_IN.Data[39].13)OTE(Axis.I.SetClock_Busy);
   113: XIC(Axis_IN.Data[39].14)OTE(Axis.I.SetClock_Error);
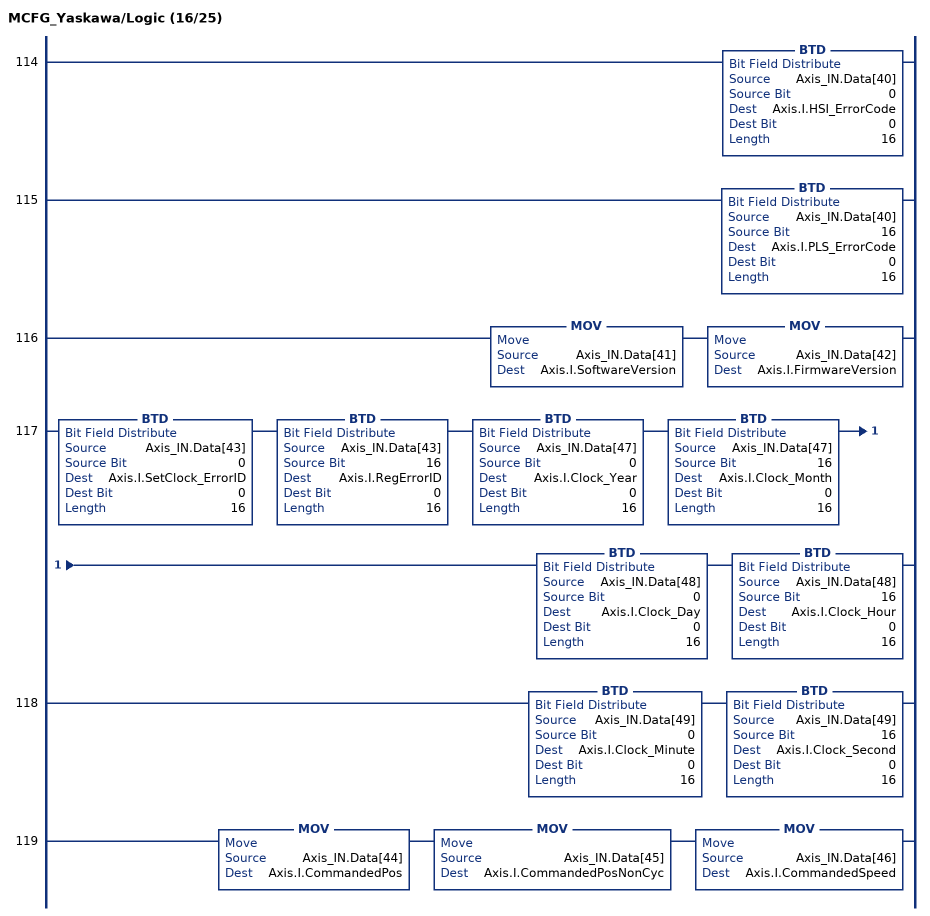
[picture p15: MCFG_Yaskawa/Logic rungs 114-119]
   114: BTD(Axis_IN.Data[40],0,Axis.I.HSI_ErrorCode,0,16);
   115: BTD(Axis_IN.Data[40],16,Axis.I.PLS_ErrorCode,0,16);
   116: MOV(Axis_IN.Data[41],Axis.I.SoftwareVersion)MOV(Axis_IN.Data[42],Axis.I.FirmwareVersion);
   117: BTD(Axis_IN.Data[43],0,Axis.I.SetClock_ErrorID,0,16)BTD(Axis_IN.Data[43],16,Axis.I.RegErrorID,0,16)BTD(Axis_IN.Data[47],0,Axis.I.Clock_Year,0,16)BTD(Axis_IN.Data[47],16,Axis.I.Clock_Month,0,16)BTD(Axis_IN.Data[48],0,Axis.I.Clock_Day,0,16)BTD(Axis_IN.Data[48],16,Axis.I.Clock_Hour,0,16);
   118: BTD(Axis_IN.Data[49],0,Axis.I.Clock_Minute,0,16)BTD(Axis_IN.Data[49],16,Axis.I.Clock_Second,0,16);
   119: MOV(Axis_IN.Data[44],Axis.I.CommandedPos)MOV(Axis_IN.Data[45],Axis.I.CommandedPosNonCyc)MOV(Axis_IN.Data[46],Axis.I.CommandedSpeed);
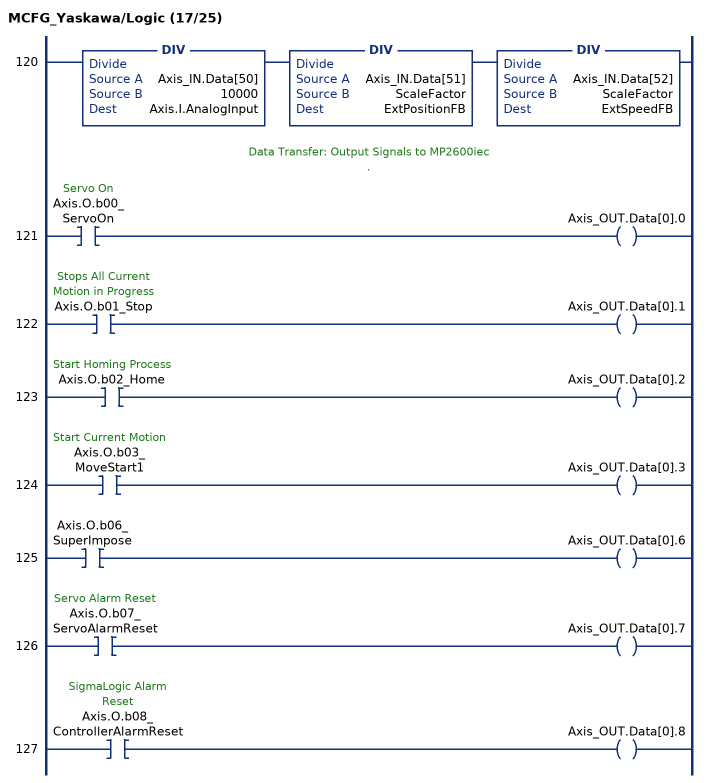
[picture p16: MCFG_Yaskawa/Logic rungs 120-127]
   120: DIV(Axis_IN.Data[50],10000,Axis.I.AnalogInput)DIV(Axis_IN.Data[51],ScaleFactor,ExtPositionFB)DIV(Axis_IN.Data[52],ScaleFactor,ExtSpeedFB);
   // Data Transfer: Output Signals to MP2600iec
   // .
   121: XIC(Axis.O.b00_ServoOn)OTE(Axis_OUT.Data[0].0);
   122: XIC(Axis.O.b01_Stop)OTE(Axis_OUT.Data[0].1);
   123: XIC(Axis.O.b02_Home)OTE(Axis_OUT.Data[0].2);
   124: XIC(Axis.O.b03_MoveStart1)OTE(Axis_OUT.Data[0].3);
   125: XIC(Axis.O.b06_SuperImpose)OTE(Axis_OUT.Data[0].6);
   126: XIC(Axis.O.b07_ServoAlarmReset)OTE(Axis_OUT.Data[0].7);
   127: XIC(Axis.O.b08_ControllerAlarmReset)OTE(Axis_OUT.Data[0].8);
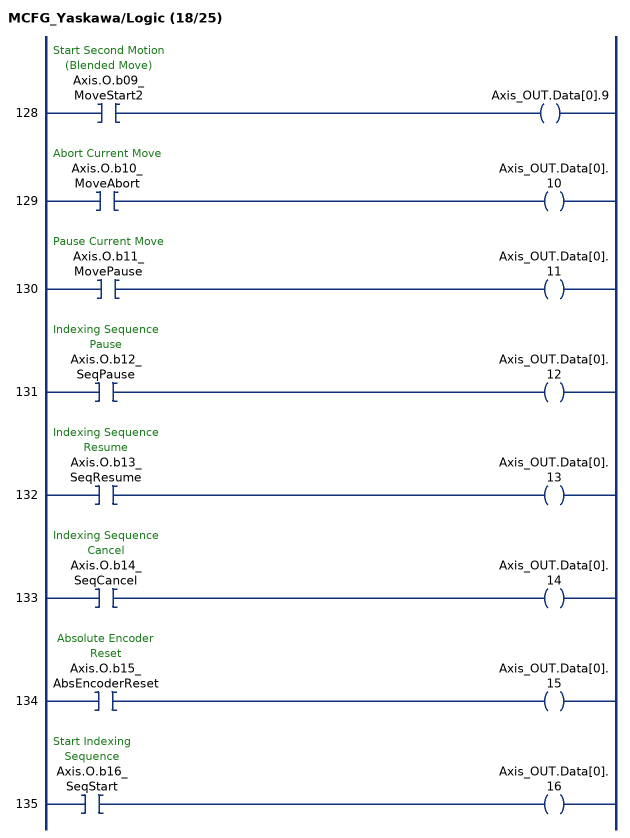
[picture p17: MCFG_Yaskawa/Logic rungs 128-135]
   128: XIC(Axis.O.b09_MoveStart2)OTE(Axis_OUT.Data[0].9);
   129: XIC(Axis.O.b10_MoveAbort)OTE(Axis_OUT.Data[0].10);
   130: XIC(Axis.O.b11_MovePause)OTE(Axis_OUT.Data[0].11);
   131: XIC(Axis.O.b12_SeqPause)OTE(Axis_OUT.Data[0].12);
   132: XIC(Axis.O.b13_SeqResume)OTE(Axis_OUT.Data[0].13);
   133: XIC(Axis.O.b14_SeqCancel)OTE(Axis_OUT.Data[0].14);
   134: XIC(Axis.O.b15_AbsEncoderReset)OTE(Axis_OUT.Data[0].15);
   135: XIC(Axis.O.b16_SeqStart)OTE(Axis_OUT.Data[0].16);
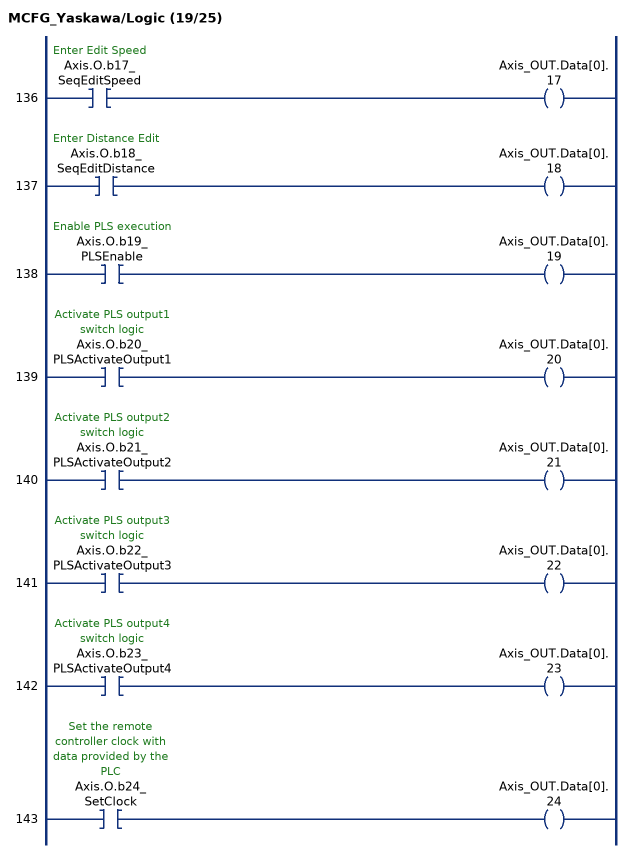
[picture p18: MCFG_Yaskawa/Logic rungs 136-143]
   136: XIC(Axis.O.b17_SeqEditSpeed)OTE(Axis_OUT.Data[0].17);
   137: XIC(Axis.O.b18_SeqEditDistance)OTE(Axis_OUT.Data[0].18);
   138: XIC(Axis.O.b19_PLSEnable)OTE(Axis_OUT.Data[0].19);
   139: XIC(Axis.O.b20_PLSActivateOutput1)OTE(Axis_OUT.Data[0].20);
   140: XIC(Axis.O.b21_PLSActivateOutput2)OTE(Axis_OUT.Data[0].21);
   141: XIC(Axis.O.b22_PLSActivateOutput3)OTE(Axis_OUT.Data[0].22);
   142: XIC(Axis.O.b23_PLSActivateOutput4)OTE(Axis_OUT.Data[0].23);
   143: XIC(Axis.O.b24_SetClock)OTE(Axis_OUT.Data[0].24);
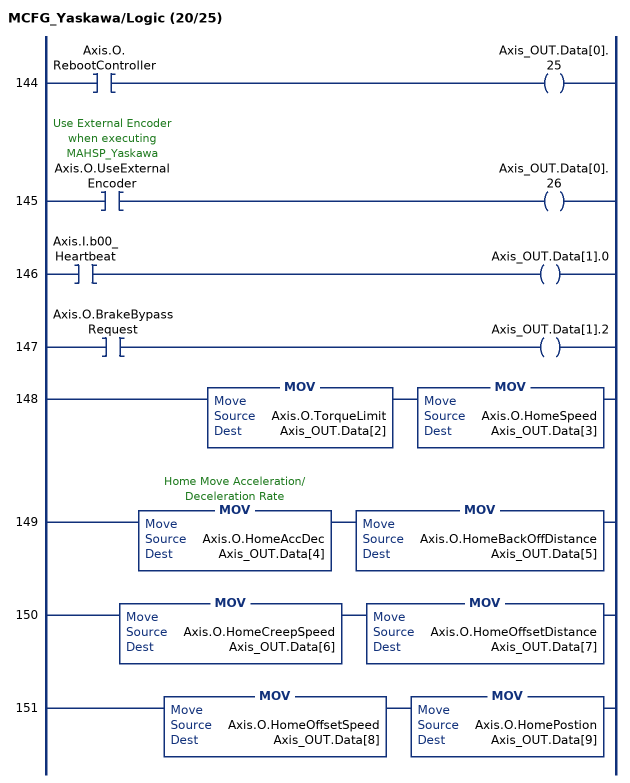
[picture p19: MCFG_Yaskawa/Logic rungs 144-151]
   144: XIC(Axis.O.RebootController)OTE(Axis_OUT.Data[0].25);
   145: XIC(Axis.O.UseExternalEncoder)OTE(Axis_OUT.Data[0].26);
   146: XIC(Axis.I.b00_Heartbeat)OTE(Axis_OUT.Data[1].0);
   147: XIC(Axis.O.BrakeBypassRequest)OTE(Axis_OUT.Data[1].2);
   148: MOV(Axis.O.TorqueLimit,Axis_OUT.Data[2])MOV(Axis.O.HomeSpeed,Axis_OUT.Data[3]);
   149: MOV(Axis.O.HomeAccDec,Axis_OUT.Data[4])MOV(Axis.O.HomeBackOffDistance,Axis_OUT.Data[5]);
   150: MOV(Axis.O.HomeCreepSpeed,Axis_OUT.Data[6])MOV(Axis.O.HomeOffsetDistance,Axis_OUT.Data[7]);
   151: MOV(Axis.O.HomeOffsetSpeed,Axis_OUT.Data[8])MOV(Axis.O.HomePostion,Axis_OUT.Data[9]);
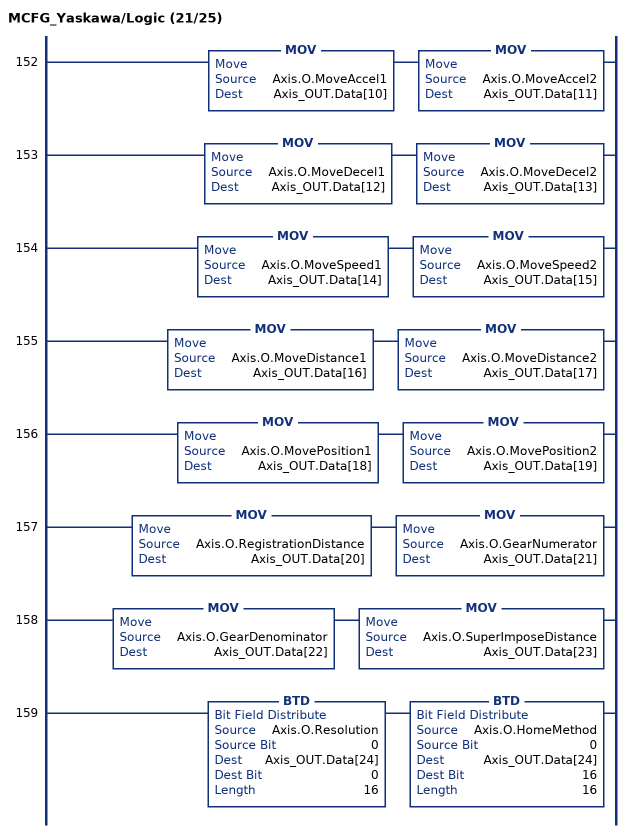
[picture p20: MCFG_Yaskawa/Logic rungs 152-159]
   152: MOV(Axis.O.MoveAccel1,Axis_OUT.Data[10])MOV(Axis.O.MoveAccel2,Axis_OUT.Data[11]);
   153: MOV(Axis.O.MoveDecel1,Axis_OUT.Data[12])MOV(Axis.O.MoveDecel2,Axis_OUT.Data[13]);
   154: MOV(Axis.O.MoveSpeed1,Axis_OUT.Data[14])MOV(Axis.O.MoveSpeed2,Axis_OUT.Data[15]);
   155: MOV(Axis.O.MoveDistance1,Axis_OUT.Data[16])MOV(Axis.O.MoveDistance2,Axis_OUT.Data[17]);
   156: MOV(Axis.O.MovePosition1,Axis_OUT.Data[18])MOV(Axis.O.MovePosition2,Axis_OUT.Data[19]);
   157: MOV(Axis.O.RegistrationDistance,Axis_OUT.Data[20])MOV(Axis.O.GearNumerator,Axis_OUT.Data[21]);
   158: MOV(Axis.O.GearDenominator,Axis_OUT.Data[22])MOV(Axis.O.SuperImposeDistance,Axis_OUT.Data[23]);
   159: BTD(Axis.O.Resolution,0,Axis_OUT.Data[24],0,16)BTD(Axis.O.HomeMethod,0,Axis_OUT.Data[24],16,16);
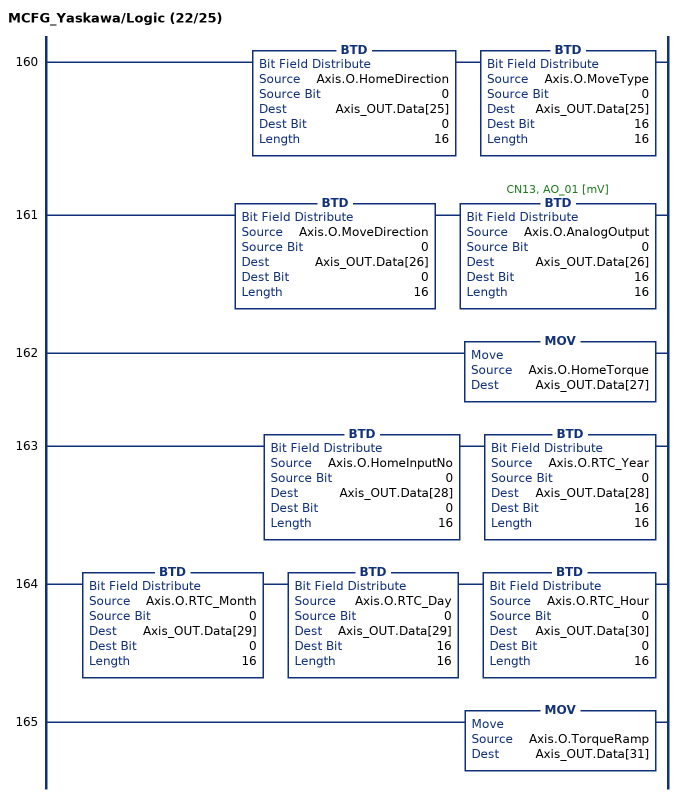
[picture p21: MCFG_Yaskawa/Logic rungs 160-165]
   160: BTD(Axis.O.HomeDirection,0,Axis_OUT.Data[25],0,16)BTD(Axis.O.MoveType,0,Axis_OUT.Data[25],16,16);
   161: BTD(Axis.O.MoveDirection,0,Axis_OUT.Data[26],0,16)BTD(Axis.O.AnalogOutput,0,Axis_OUT.Data[26],16,16);
   162: MOV(Axis.O.HomeTorque,Axis_OUT.Data[27]);
   163: BTD(Axis.O.HomeInputNo,0,Axis_OUT.Data[28],0,16)BTD(Axis.O.RTC_Year,0,Axis_OUT.Data[28],16,16);
   164: BTD(Axis.O.RTC_Month,0,Axis_OUT.Data[29],0,16)BTD(Axis.O.RTC_Day,0,Axis_OUT.Data[29],16,16)BTD(Axis.O.RTC_Hour,0,Axis_OUT.Data[30],0,16);
   165: MOV(Axis.O.TorqueRamp,Axis_OUT.Data[31]);
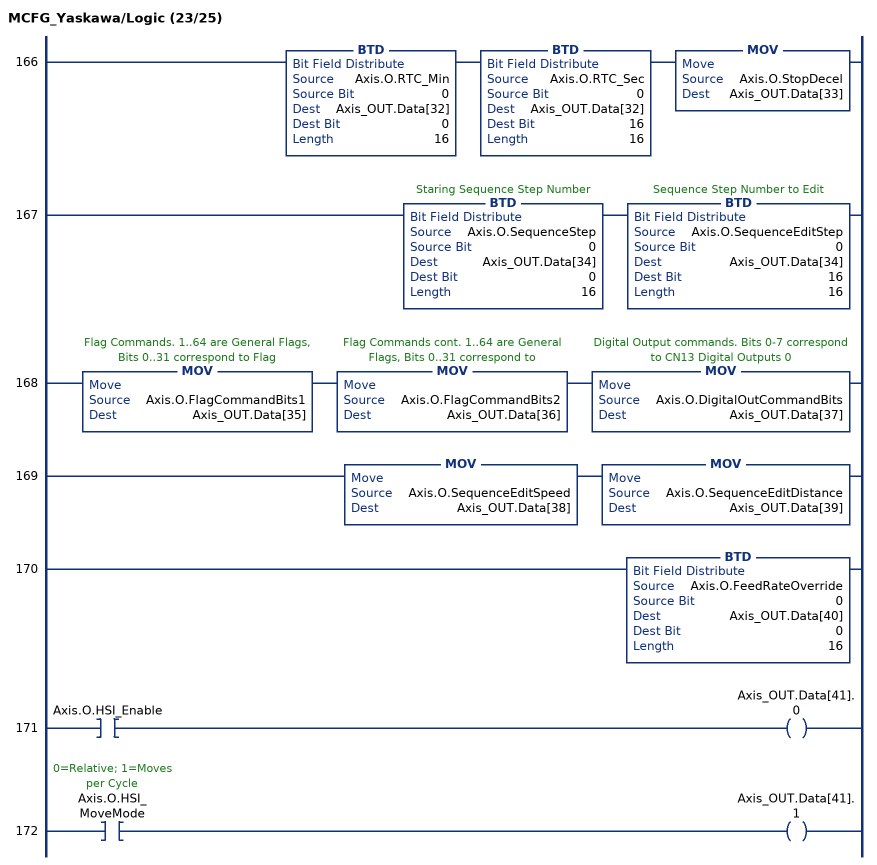
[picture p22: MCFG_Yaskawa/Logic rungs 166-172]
   166: BTD(Axis.O.RTC_Min,0,Axis_OUT.Data[32],0,16)BTD(Axis.O.RTC_Sec,0,Axis_OUT.Data[32],16,16)MOV(Axis.O.StopDecel,Axis_OUT.Data[33]);
   167: BTD(Axis.O.SequenceStep,0,Axis_OUT.Data[34],0,16)BTD(Axis.O.SequenceEditStep,0,Axis_OUT.Data[34],16,16);
   168: MOV(Axis.O.FlagCommandBits1,Axis_OUT.Data[35])MOV(Axis.O.FlagCommandBits2,Axis_OUT.Data[36])MOV(Axis.O.DigitalOutCommandBits,Axis_OUT.Data[37]);
   169: MOV(Axis.O.SequenceEditSpeed,Axis_OUT.Data[38])MOV(Axis.O.SequenceEditDistance,Axis_OUT.Data[39]);
   170: BTD(Axis.O.FeedRateOverride,0,Axis_OUT.Data[40],0,16);
   171: XIC(Axis.O.HSI_Enable)OTE(Axis_OUT.Data[41].0);
   172: XIC(Axis.O.HSI_MoveMode)OTE(Axis_OUT.Data[41].1);
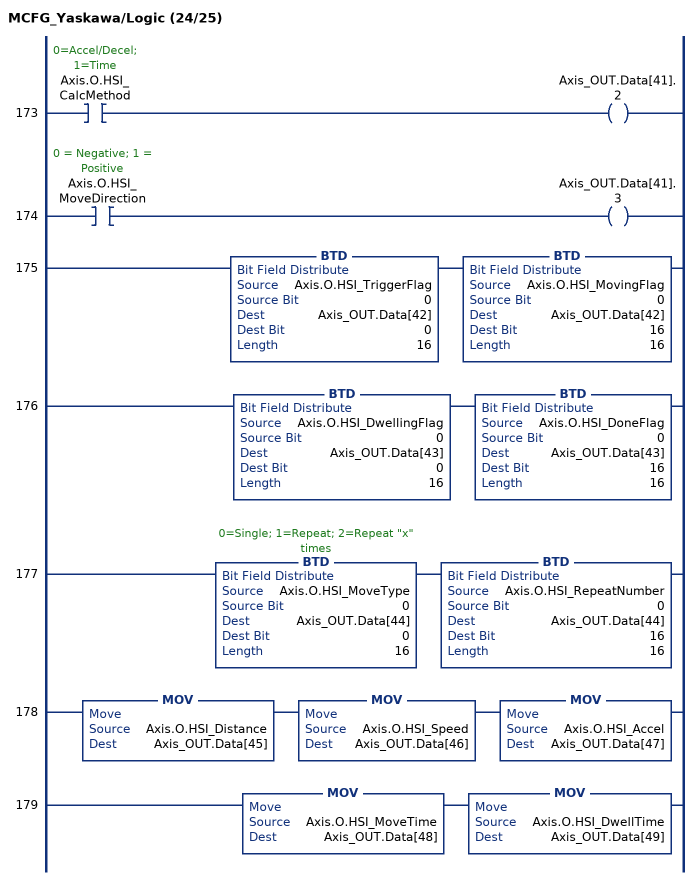
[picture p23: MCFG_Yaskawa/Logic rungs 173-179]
   173: XIC(Axis.O.HSI_CalcMethod)OTE(Axis_OUT.Data[41].2);
   174: XIC(Axis.O.HSI_MoveDirection)OTE(Axis_OUT.Data[41].3);
   175: BTD(Axis.O.HSI_TriggerFlag,0,Axis_OUT.Data[42],0,16)BTD(Axis.O.HSI_MovingFlag,0,Axis_OUT.Data[42],16,16);
   176: BTD(Axis.O.HSI_DwellingFlag,0,Axis_OUT.Data[43],0,16)BTD(Axis.O.HSI_DoneFlag,0,Axis_OUT.Data[43],16,16);
   177: BTD(Axis.O.HSI_MoveType,0,Axis_OUT.Data[44],0,16)BTD(Axis.O.HSI_RepeatNumber,0,Axis_OUT.Data[44],16,16);
   178: MOV(Axis.O.HSI_Distance,Axis_OUT.Data[45])MOV(Axis.O.HSI_Speed,Axis_OUT.Data[46])MOV(Axis.O.HSI_Accel,Axis_OUT.Data[47]);
   179: MOV(Axis.O.HSI_MoveTime,Axis_OUT.Data[48])MOV(Axis.O.HSI_DwellTime,Axis_OUT.Data[49]);
